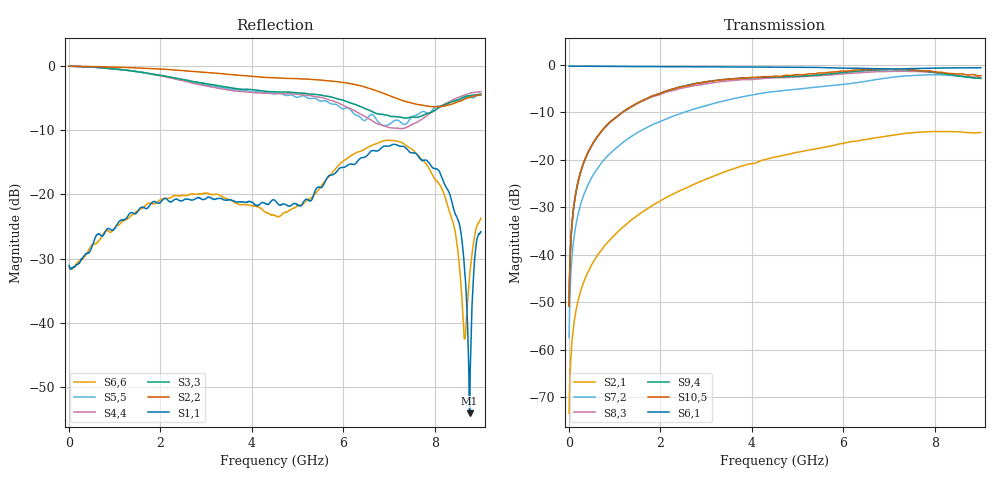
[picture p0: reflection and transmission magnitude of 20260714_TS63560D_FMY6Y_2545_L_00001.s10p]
# GHz S DB R 50
! CMT, SN0916, 25263762, 26.7.0
! Date: 15.07.2026 13:18:10
! Data: Format
! Freq S1.1:dB/Ang S1.2:dB/Ang S1.3:dB/Ang S1.4:dB/Ang S1.5:dB/Ang S1.6:dB/Ang S1.7:dB/Ang S1.8:dB/Ang S1.9:dB/Ang S1.10:dB/Ang
!  S2.1:dB/Ang S2.2:dB/Ang S2.3:dB/Ang S2.4:dB/Ang S2.5:dB/Ang S2.6:dB/Ang S2.7:dB/Ang S2.8:dB/Ang S2.9:dB/Ang S2.10:dB/Ang
!  S3.1:dB/Ang S3.2:dB/Ang S3.3:dB/Ang S3.4:dB/Ang S3.5:dB/Ang S3.6:dB/Ang S3.7:dB/Ang S3.8:dB/Ang S3.9:dB/Ang S3.10:dB/Ang
!  S4.1:dB/Ang S4.2:dB/Ang S4.3:dB/Ang S4.4:dB/Ang S4.5:dB/Ang S4.6:dB/Ang S4.7:dB/Ang S4.8:dB/Ang S4.9:dB/Ang S4.10:dB/Ang
!  S5.1:dB/Ang S5.2:dB/Ang S5.3:dB/Ang S5.4:dB/Ang S5.5:dB/Ang S5.6:dB/Ang S5.7:dB/Ang S5.8:dB/Ang S5.9:dB/Ang S5.10:dB/Ang
!  S6.1:dB/Ang S6.2:dB/Ang S6.3:dB/Ang S6.4:dB/Ang S6.5:dB/Ang S6.6:dB/Ang S6.7:dB/Ang S6.8:dB/Ang S6.9:dB/Ang S6.10:dB/Ang
!  S7.1:dB/Ang S7.2:dB/Ang S7.3:dB/Ang S7.4:dB/Ang S7.5:dB/Ang S7.6:dB/Ang S7.7:dB/Ang S7.8:dB/Ang S7.9:dB/Ang S7.10:dB/Ang
!  S8.1:dB/Ang S8.2:dB/Ang S8.3:dB/Ang S8.4:dB/Ang S8.5:dB/Ang S8.6:dB/Ang S8.7:dB/Ang S8.8:dB/Ang S8.9:dB/Ang S8.10:dB/Ang
!  S9.1:dB/Ang S9.2:dB/Ang S9.3:dB/Ang S9.4:dB/Ang S9.5:dB/Ang S9.6:dB/Ang S9.7:dB/Ang S9.8:dB/Ang S9.9:dB/Ang S9.10:dB/Ang
!  S10.1:dB/Ang S10.2:dB/Ang S10.3:dB/Ang S10.4:dB/Ang S10.5:dB/Ang S10.6:dB/Ang S10.7:dB/Ang S10.8:dB/Ang S10.9:dB/Ang S10.10:dB/Ang
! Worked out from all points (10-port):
!   2001 points, 10 MHz to 9 GHz, reference 50 ohm
!   strongest paths, dB at 10 MHz, 2.257 GHz, 4.505 GHz, 6.753 GHz, 9 GHz:
!     S6,1: -0.3, -0.4, -0.5, -0.8, -0.6
!     S10,5: -50.8, -5.1, -2.3, -0.8, -2.2
!     S9,4: -50.9, -5.1, -2.5, -1.0, -2.8
!     S8,3: -50.7, -5.4, -2.7, -1.4, -2.6
!     S7,2: -57.4, -10.9, -5.6, -3.0, -2.7
!     S2,1: -73.4, -27.3, -19.4, -15.3, -14.2
!   lowest |S11| = -54.1 dB at 8.753 GHz (marker M1), VSWR 1.00, Z = 50 - j0.197 ohm
!   |S11| at or under -10 dB: start of sweep to end of sweep
